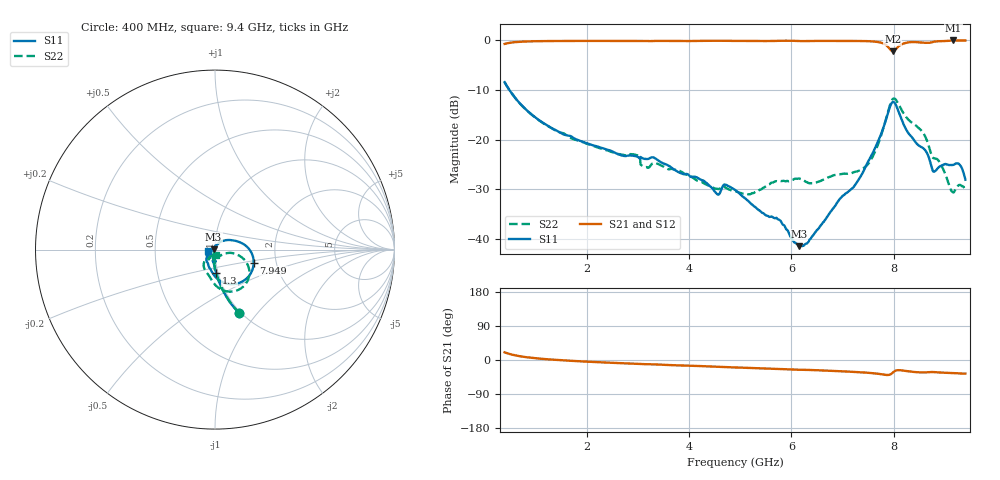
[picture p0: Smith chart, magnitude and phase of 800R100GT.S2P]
!  American Technical Ceramics  Date:  6/19/09
!  One Norden Lane
!  Huntington Station,  NY.  11746-2102
!  Tel:  (631) 622-4700  Fax:  (631) 622-4748
!  Part Number  800R100GT
!  Description: Ultra-low ESR, NPO  Mounting Orientation: Vertical
!  Application: High RF power Filters, Combiners, Matching networks,
!  Antenna, DC block, Bypass and Couplers
# GHZ S DB R 50
! Freq  |S11|  S11 Ph  |S21|  S21 Ph  |S12|  S12 Ph  |S22|  S22 Ph
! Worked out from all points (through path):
!   801 points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, 400 MHz to 9.4 GHz, reference 50 ohm
!   highest |S21| = -0.01 dB at 9.164 GHz (marker M1); lowest = -2.2 dB at 7.983 GHz (marker M2)
!   group delay of S21, straight-line fit = 14 ps
!   lowest |S11| = -41.5 dB at 6.149 GHz (marker M3), VSWR 1.02, Z = 49.2 + j0.184 ohm
!   |S11| at or under -10 dB: 494.3 MHz to end of sweep
!   |S22| runs from -31.1 to -8.4 dB; largest |S21 - S12| = 0.0029
!   S11 on the Smith chart (normalised r, x): 400 MHz: 0.98, -0.81; 1.3 GHz: 0.98, -0.26; 7.949 GHz: 1.53, -0.24; 9.4 GHz: 0.93, -0.01
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0.4  -8.42 -69.1  -0.71 20.3  -0.72 20.3  -8.43 -69.1
1.3  -17.56 -87.0  -0.12 1.3  -0.13 1.3  -17.59 -87.0
1.908  -20.36 -91.2  -0.10 -3.6  -0.10 -3.6  -20.43 -90.8
2.988  -23.41 -99.0  -0.11 -10.1  -0.11 -10.0  -23.14 -94.4
3.156  -23.88 -87.1  -0.11 -11.1  -0.12 -11.0  -25.54 -96.5
3.404  -24.20 -92.4  -0.09 -12.0  -0.09 -12.0  -24.94 -99.5
4.551  -30.99 -85.3  -0.06 -17.8  -0.06 -17.7  -29.93 -96.3
4.709  -29.06 -82.0  -0.08 -18.8  -0.08 -18.7  -29.66 -94.8
4.9  -30.15 -91.5  -0.10 -19.6  -0.10 -19.6  -30.39 -90.2
5.755  -36.11 -118.1  -0.09 -23.3  -0.09 -23.2  -28.32 -67.3
6.149  -41.48 167.2  -0.12 -25.7  -0.12 -25.6  -27.81 -67.6
6.408  -39.51 118.0  -0.12 -26.5  -0.12 -26.4  -28.80 -62.3
7.465  -25.16 54.5  -0.15 -33.3  -0.15 -33.2  -25.30 -26.8
7.668  -20.96 36.8  -0.29 -35.9  -0.28 -35.8  -21.65 -12.7
7.904  -14.08 -2.2  -1.48 -39.4  -1.47 -39.3  -13.85 -25.4
7.949  -12.84 -18.9  -2.01 -36.9  -2.00 -36.8  -12.40 -37.5
7.983  -12.42 -33.5  -2.19 -33.2  -2.18 -33.2  -11.80 -48.7
8.196  -16.99 -92.6  -0.62 -28.2  -0.61 -28.1  -14.77 -93.2
8.568  -21.68 -121.9  -0.44 -32.8  -0.43 -32.8  -18.54 -121.0
8.781  -26.48 -127.7  -0.27 -31.9  -0.26 -31.8  -23.75 -123.8
9.164  -25.10 -132.5  -0.01 -34.2  -0.01 -34.1  -30.66 -100.2
9.4  -28.08 -168.6  -0.01 -35.9  -0.01 -35.8  -30.06 -83.2
